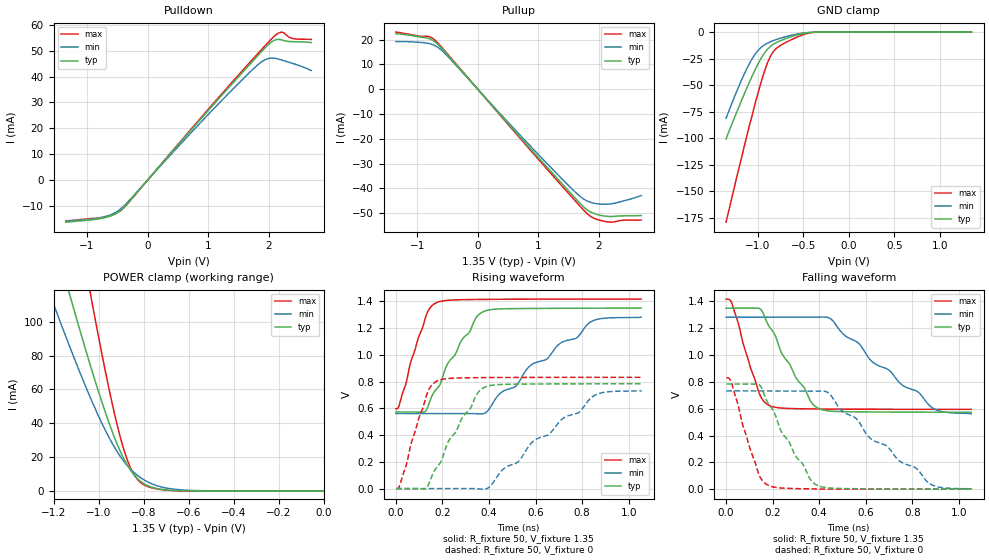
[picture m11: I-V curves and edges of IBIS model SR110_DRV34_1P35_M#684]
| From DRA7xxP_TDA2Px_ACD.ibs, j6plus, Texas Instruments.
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| Model based on original model for DDR_DIFFIOPB_H
|   Sub model SR110_DRV34_1P35
[model]   SR110_DRV34_1P35_M#684
|[Description]  [1.35V-I/O-X-X]
|   , ,
|[Input Load]
|[Output Drive]
|Voltage   1.35V
|Mode   I/O
Model_type   I/O
Polarity   Non-Inverting
Enable   Active-Low
Vinl =  0.585
Vinh =  0.765
Cref =  15.0000pF
Rref =  100.0000M
Vref =  0V
Vmeas =  0.675
C_comp   2p   2p   2p
[Model Spec]
Vinl   0.585   0.55125   0.61875
Vinh   0.765   0.73125   0.79875
[Receiver Thresholds]
Tslew_ac = 5n
Vth = 0.675
Vth_max = 0.709
Vth_min = 0.608
Vinh_ac = 0.175
Vinh_dc = 0.1
Vinl_ac = -0.175
Vinl_dc = -0.1
[Temperature Range]   25   125   -40
[Voltage Range]   1.35   1.2825   1.4175
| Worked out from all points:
|   slope of the pulldown table from 0 to 0.203 V, typ, clamps not added: 36.8 ohm
|   slope of the pullup table from 0 to 0.203 V, typ, clamps not added: 36 ohm
|   GND clamp passes 1 mA (typ) near -0.48 V on its own axis
|   POWER clamp passes 1 mA (typ) near -0.72 V on its own axis
|   rising waveform, R_fixture 50, V_fixture 1.35: 20-80 % time 156ps typ, 340ps min, 84ps max; typ from 0.573 V to 1.35 V
|   rising waveform, R_fixture 50, V_fixture 0: 20-80 % time 153ps typ, 334ps min, 83.2ps max; typ from 0 V to 0.784 V
|   falling waveform, R_fixture 50, V_fixture 1.35: 20-80 % time 151ps typ, 320ps min, 83.9ps max; typ from 1.35 V to 0.573 V
|   falling waveform, R_fixture 50, V_fixture 0: 20-80 % time 153ps typ, 326ps min, 84.1ps max; typ from 0.784 V to 0 V
[POWER_clamp]
-1.35V    224.4mA    165.8mA    358.5mA
-1.214V   157mA      115.5mA    250.8mA
-1.132V   117.8mA    86.59mA    187.7mA
-1.118V   111.4mA    81.92mA    177.3mA
-1.036V   74.26mA    55.16mA    116.8mA
-954.5mV  40.7mA     31.91mA    61.06mA
-900mV    22.42mA    19.79mA    30.14mA
-859.1mV  12.48mA    13.09mA    13.96mA
-804.5mV  4.85mA     7.084mA    4.132mA
-736.4mV  1.313mA    2.9mA      1.073mA
-627.3mV  101.6uA    577.3uA    45.9uA
0V        75.63nA    322.4nA    418.5nA
[Pulldown]
-1.35V    -16.25mA   -15.93mA   -15.81mA
-736.4mV  -14.67mA   -14.31mA   -14.33mA
-531.8mV  -13.09mA   -12.54mA   -12.91mA
-409.1mV  -10.94mA   -10.36mA   -11.07mA
1.145V    30.69mA    28.89mA    31.23mA
1.718V    45.54mA    42.37mA    46.27mA
1.923V    50.72mA    46.33mA    51.51mA
2.086V    53.98mA    47.12mA    55.52mA
2.209V    54.19mA    46.41mA    57.19mA
2.25V     53.89mA    46.1mA     56.9mA
2.373V    53.5mA     45.23mA    54.8mA
2.7V      53.13mA    42.33mA    54.36mA
[Pullup]
-1.35V    22.33mA    19.2mA     23.01mA
-981.8mV  21.15mA    18.91mA    21.43mA
-818.2mV  20.5mA     18.48mA    21.31mA
-736.4mV  19.62mA    17.88mA    20.36mA
-613.6mV  16.97mA    16.06mA    17.42mA
1.064V    -29.25mA   -27.93mA   -29.99mA
1.555V    -42.46mA   -40.17mA   -43.52mA
1.759V    -47.7mA    -44.45mA   -49.03mA
1.923V    -50.14mA   -45.98mA   -52.07mA
2.127V    -51.21mA   -46.35mA   -53.42mA
2.291V    -51.16mA   -45.77mA   -53.24mA
2.7V      -50.91mA   -42.85mA   -52.71mA
[GND_clamp]
-1.35V    -100.7mA   -81.27mA   -179.3mA
-1.241V   -77.31mA   -57.61mA   -140mA
-1.132V   -54.83mA   -36.31mA   -101.6mA
-1.05V    -39.08mA   -23.36mA   -74mA
-968.2mV  -25.28mA   -14.71mA   -48.34mA
-913.6mV  -18.13mA   -11.32mA   -33.52mA
-859.1mV  -13.28mA   -9.024mA   -22.35mA
-831.8mV  -11.61mA   -8.091mA   -18.64mA
-777.3mV  -9.078mA   -6.444mA   -14.07mA
-531.8mV  -1.871mA   -1.307mA   -3.441mA
-368.2mV  -88.76uA   -111.2uA   -158uA
1.35V     75.63nA    385.5nA    349.4nA
[Ramp]
dV/dt_f 0.46683908/0.15119162n 0.43396865/0.32078806n 0.49362269/84.021895p
dV/dt_r  0.4729405/0.15437158n 0.44234074/0.33552799n 0.50132504/83.661449p
R_load = 50
[Rising Waveform]
R_fixture = 50
V_fixture = 1.35
V_fixture_min = 1.2825
V_fixture_max = 1.4175
0s        573.3mV    561.4mV    596.4mV
13.62ps   573.3mV    561.3mV    620.8mV
124.2ps   574.4mV    561.3mV    1.263V
174.9ps   745.6mV    561.4mV    1.391V
281ps     1.106V     561.1mV    1.413V
379.2ps   1.326V     562.2mV    1.415V
575.4ps   1.347V     917.1mV    1.417V
777.6ps   1.349V     1.129V     1.417V
836.5ps   1.349V     1.247V     1.417V
1.053ns   1.35V      1.282V     1.417V
[Rising Waveform]
R_fixture = 50
V_fixture = 0
V_fixture_min = 0
V_fixture_max = 0
1.656ps   0V         0V         0V
17.66ps   0V         0V         30.87mV
129.6ps   0V         0V         687.2mV
177.1ps   162.7mV    0V         804.9mV
285.8ps   532.6mV    0V         828mV
384.5ps   760.3mV    -3.355mV   830.1mV
526.9ps   781.2mV    204mV      831.4mV
588.4ps   782mV      352mV      831.6mV
850.2ps   783.7mV    693.9mV    832.1mV
1.054ns   784.4mV    732.7mV    832.1mV
[Falling Waveform]
R_fixture = 50
V_fixture = 1.35
V_fixture_min = 1.2825
V_fixture_max = 1.4175
0s        1.35V      1.282V     1.417V
26.17ps   1.35V      1.283V     1.381V
143.5ps   1.347V     1.283V     710.8mV
185.8ps   1.212V     1.283V     624.3mV
301.5ps   827.7mV    1.282V     600.4mV
401ps     599.4mV    1.284V     598.1mV
451.5ps   581.9mV    1.268V     597.4mV
628.6ps   575.8mV    950.1mV    596.2mV
888.7ps   574.1mV    603.8mV    595.8mV
1.053ns   573.3mV    561.4mV    595.7mV
[Falling Waveform]
R_fixture = 50
V_fixture = 0
V_fixture_min = 0
V_fixture_max = 0
1.656ps   784.4mV    732.7mV    831.2mV
23.31ps   784.5mV    732.7mV    794mV
140.2ps   780.5mV    732.8mV    113.1mV
182.8ps   635.5mV    732.7mV    27.52mV
297.9ps   249.6mV    732.6mV    4.244mV
395.1ps   26.11mV    733.2mV    0V
441.8ps   9.013mV    715.3mV    0V
617ps     2.282mV    383mV      0V
874.9ps   0V         40.93mV    0V
1.054ns   0V         0V         0V
